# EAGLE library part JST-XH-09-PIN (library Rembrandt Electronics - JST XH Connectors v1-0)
JST XH Connector 2 Pin Wire to board connector. Pitch: 2,54 mm, (0.100") Number of pins: 9 Created by Rembrandt Electronics www.rembrandtelectronics.com
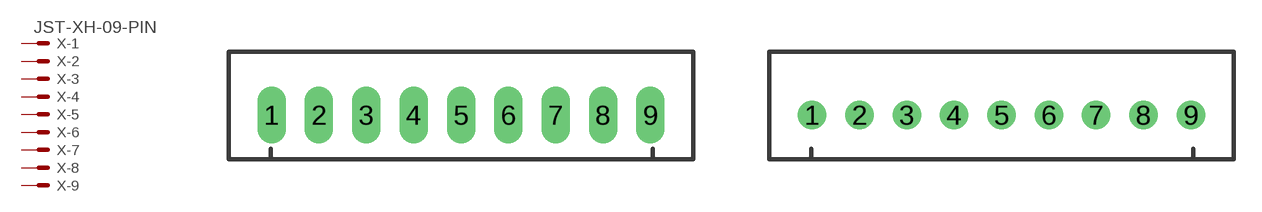
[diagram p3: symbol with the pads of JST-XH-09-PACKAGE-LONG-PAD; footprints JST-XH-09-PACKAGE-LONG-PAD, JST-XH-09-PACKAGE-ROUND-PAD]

Designator prefix X; gates -1=MV -2=M -3=M -4=M -5=M -6=M -7=M -8=M -9=M

## JST-XH-09-PIN-LONG-PAD  [JST-XH-09-PACKAGE-LONG-PAD]
1  -1:S  pas
2  -2:S  pas
3  -3:S  pas
4  -4:S  pas
5  -5:S  pas
6  -6:S  pas
7  -7:S  pas
8  -8:S  pas
9  -9:S  pas

## JST-XH-09-PIN-ROUND-PAD  [JST-XH-09-PACKAGE-ROUND-PAD]
Pads as for JST-XH-09-PACKAGE-LONG-PAD

## Footprint JST-XH-09-PACKAGE-LONG-PAD (pad centres in mm)
JST XH Connector Long Pads (Package) Wire to board connector. Pitch: 2,54 mm, (0.100") Number of pins: 9 Created by Rembrandt Electronics www.rembrandtelectronics.com
drill 1.016 long: 1 -10.16,0; 2 -7.62,0; 3 -5.08,0; 4 -2.54,0; 5 0,0; 6 2.54,0; 7 5.08,0; 8 7.62,0; 9 10.16,0

## Footprint JST-XH-09-PACKAGE-ROUND-PAD (pad centres in mm)
JST XH Connector Round Pads (Package) Wire to board connector. Pitch: 2,54 mm, (0.100") Number of pins: 9 Created by Rembrandt Electronics www.rembrandtelectronics.com
drill 1.016: 1 -10.16,0; 2 -7.62,0; 3 -5.08,0; 4 -2.54,0; 5 0,0; 6 2.54,0; 7 5.08,0; 8 7.62,0; 9 10.16,0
